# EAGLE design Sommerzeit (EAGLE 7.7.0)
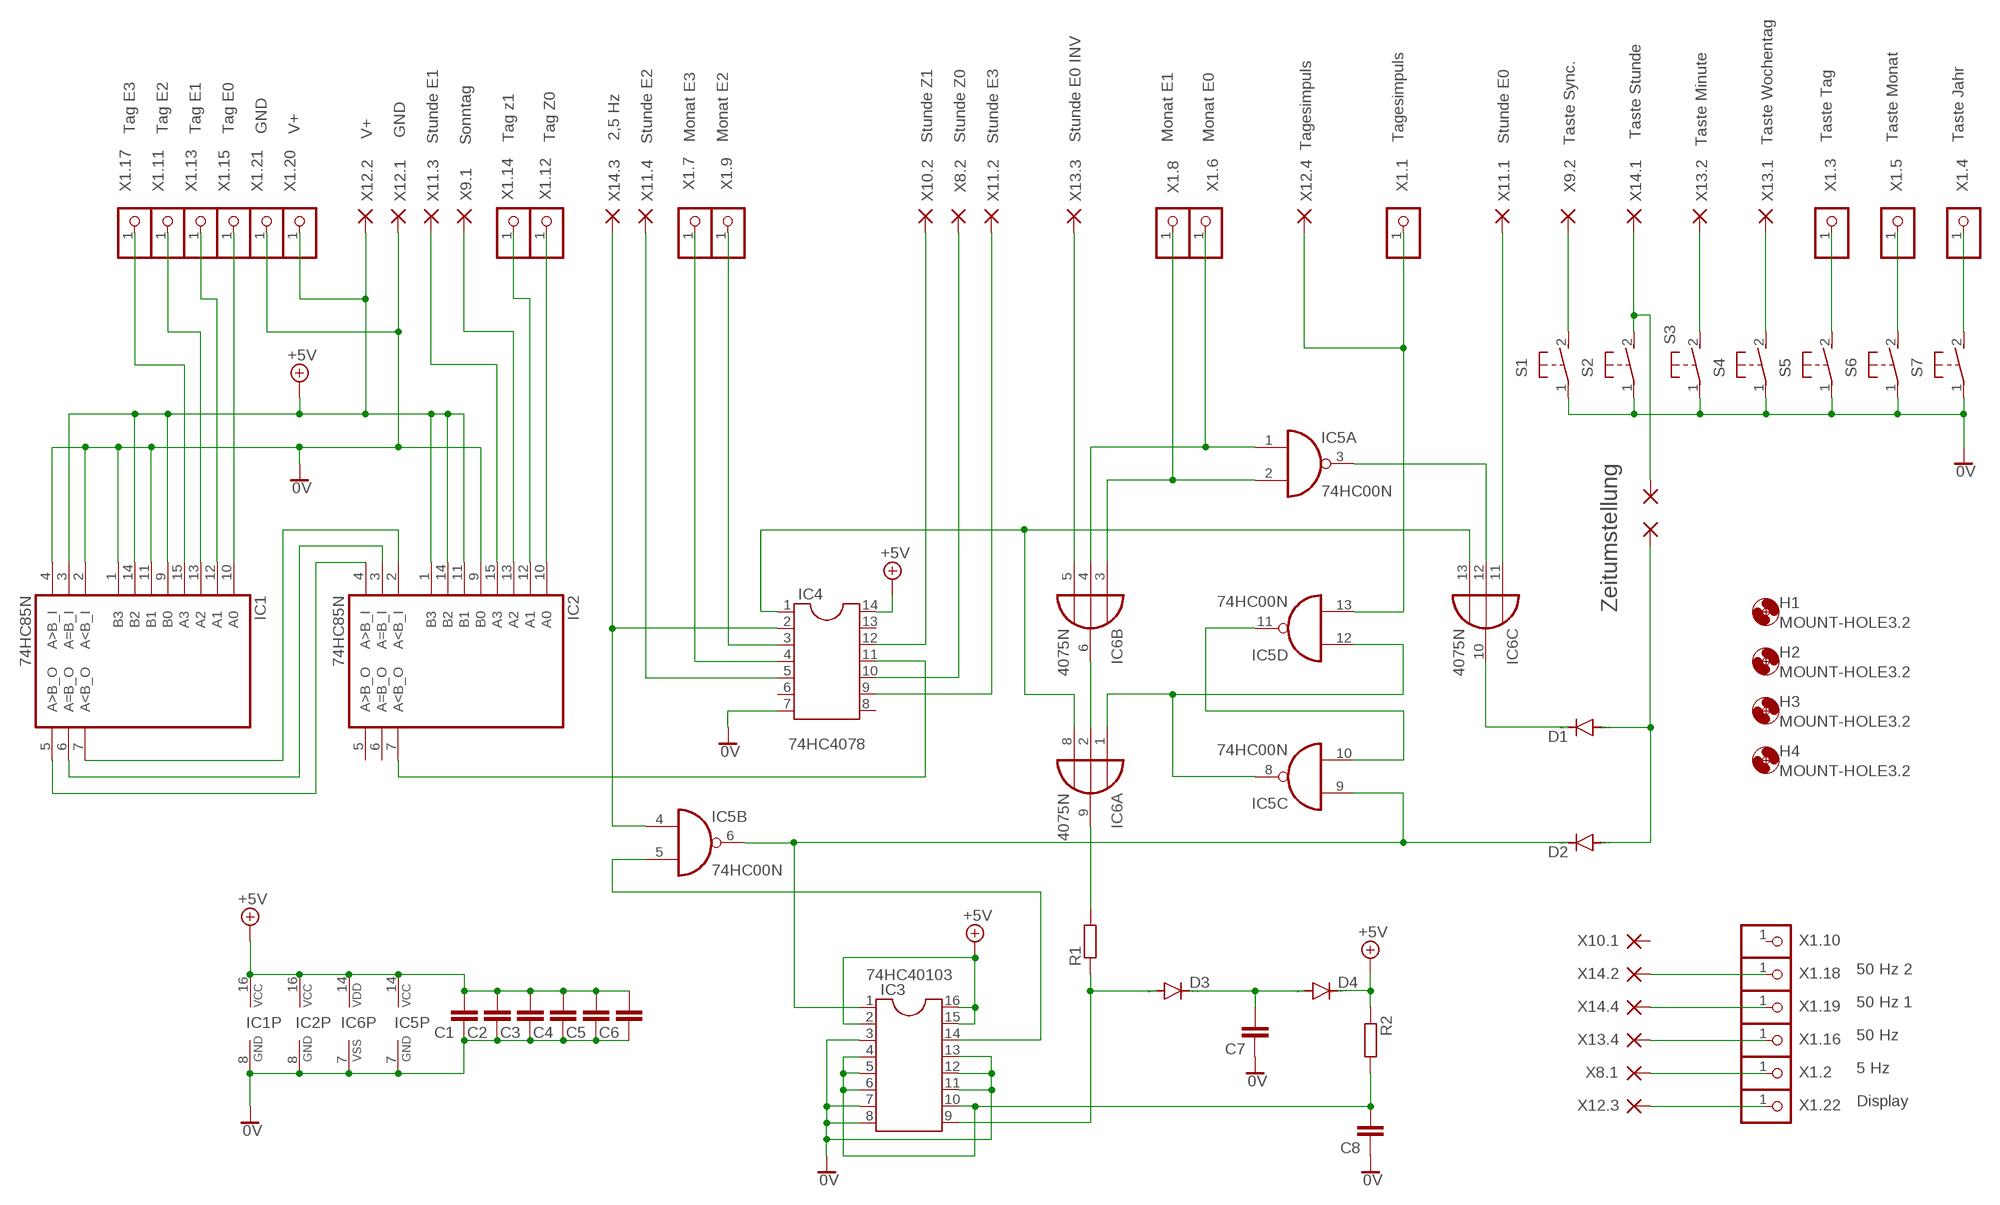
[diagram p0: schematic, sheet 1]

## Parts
C1  C-EU050-024X044  [C050-024X044]
C2  C-EU050-024X044  [C050-024X044]
C3  C-EU050-024X044  [C050-024X044]
C4  C-EU050-024X044  [C050-024X044]
C5  C-EU050-024X044  [C050-024X044]
C6  C-EU050-024X044  [C050-024X044]
C7  C-EU050-024X044  [C050-024X044]
C8  C-EU050-024X044  [C050-024X044]
D1  1N4148DO35-10  [DO35-10]
D2  1N4148DO35-10  [DO35-10]
D3  1N4148DO35-10  [DO35-10]
D4  1N4148DO35-10  [DO35-10]
H1  MOUNT-HOLE3.2  [3,2]
H2  MOUNT-HOLE3.2  [3,2]
H3  MOUNT-HOLE3.2  [3,2]
H4  MOUNT-HOLE3.2  [3,2]
IC1  74HC85N  [DIL16]
IC2  74HC85N  [DIL16]
IC3  DIL16  [DIL16]
IC4  DIL14  [DIL14]
IC5  74HC00N  [DIL14]
IC6  4075N  [DIL14]
PAD1  WIREPAD1,6/0,8  [1,6/0,8]
PAD2  WIREPAD1,6/0,8  [1,6/0,8]
R1  R-EU_0207/10  [0207/10]
R2  R-EU_0207/10  [0207/10]
S1  31-XX  [B3F-31XX]
S2  31-XX  [B3F-31XX]
S3  31-XX  [B3F-31XX]
S4  31-XX  [B3F-31XX]
S5  31-XX  [B3F-31XX]
S6  31-XX  [B3F-31XX]
S7  31-XX  [B3F-31XX]
X1.1  Tagesimpuls  PINHD-1X1  [1X01]
X1.2  5 Hz  PINHD-1X1  [1X01]
X1.3  Taste Tag  PINHD-1X1  [1X01]
X1.4  Taste Jahr  PINHD-1X1  [1X01]
X1.5  Taste Monat  PINHD-1X1  [1X01]
X1.6  Monat E0  PINHD-1X1  [1X01]
X1.7  Monat E3  PINHD-1X1  [1X01]
X1.8  Monat E1  PINHD-1X1  [1X01]
X1.9  Monat E2  PINHD-1X1  [1X01]
X1.10  PINHD-1X1  [1X01]
X1.11  Tag E2  PINHD-1X1  [1X01]
X1.12  Tag Z0  PINHD-1X1  [1X01]
X1.13  Tag E1  PINHD-1X1  [1X01]
X1.14  Tag z1  PINHD-1X1  [1X01]
X1.15  Tag E0  PINHD-1X1  [1X01]
X1.16  50 Hz  PINHD-1X1  [1X01]
X1.17  Tag E3  PINHD-1X1  [1X01]
X1.18  50 Hz 2  PINHD-1X1  [1X01]
X1.19  50 Hz 1  PINHD-1X1  [1X01]
X1.20  V+  PINHD-1X1  [1X01]
X1.21  GND  PINHD-1X1  [1X01]
X1.22  Display  PINHD-1X1  [1X01]
X8.1  WIREPAD1,6/0,8  [1,6/0,8]
X8.2  Stunde Z0  WIREPAD1,6/0,8  [1,6/0,8]
X9.1  Sonntag  WIREPAD1,6/0,8  [1,6/0,8]
X9.2  Taste Sync.  WIREPAD1,6/0,8  [1,6/0,8]
X10.1  WIREPAD1,6/0,8  [1,6/0,8]
X10.2  Stunde Z1  WIREPAD1,6/0,8  [1,6/0,8]
X11.1  Stunde E0  WIREPAD1,6/0,8  [1,6/0,8]
X11.2  Stunde E3  WIREPAD1,6/0,8  [1,6/0,8]
X11.3  Stunde E1  WIREPAD1,6/0,8  [1,6/0,8]
X11.4  Stunde E2  WIREPAD1,6/0,8  [1,6/0,8]
X12.1  GND  WIREPAD1,6/0,8  [1,6/0,8]
X12.2  V+  WIREPAD1,6/0,8  [1,6/0,8]
X12.3  WIREPAD1,6/0,8  [1,6/0,8]
X12.4  Tagesimpuls  WIREPAD1,6/0,8  [1,6/0,8]
X13.1  Taste Wochentag  WIREPAD1,6/0,8  [1,6/0,8]
X13.2  Taste Minute  WIREPAD1,6/0,8  [1,6/0,8]
X13.3  Stunde E0 INV  WIREPAD1,6/0,8  [1,6/0,8]
X13.4  WIREPAD1,6/0,8  [1,6/0,8]
X14.1  Taste Stunde  WIREPAD1,6/0,8  [1,6/0,8]
X14.2  WIREPAD1,6/0,8  [1,6/0,8]
X14.3  2,5 Hz  WIREPAD1,6/0,8  [1,6/0,8]
X14.4  WIREPAD1,6/0,8  [1,6/0,8]

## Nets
0V: C1.1 C2.1 C3.1 C4.1 C5.1 C6.1 C7.1 C8.1 IC1.1(B3) IC1.2(A<B_I) IC1.4(A>B_I) IC1.8(GND) IC1.11(B1) IC2.8(GND) IC2.9(B0) IC3.3 IC3.7 IC3.8 IC3.11 IC3.12 IC3.13 IC4.7 IC5.7(P:GND) IC6.7(P:VSS) S1.1(P) S2.1(P) S3.1(P) S4.1(P) S5.1(P) S6.1(P) S7.1(P) X1.21.1 X12.1.1(P)
+5V: C1.2 C2.2 C3.2 C4.2 C5.2 C6.2 D4.C IC1.3(A=B_I) IC1.9(B0) IC1.14(B2) IC1.16(VCC) IC2.1(B3) IC2.11(B1) IC2.14(B2) IC2.16(VCC) IC3.2 IC3.15 IC3.16 IC4.14 IC5.14(P:VCC) IC6.14(P:VDD) R2.1 X1.20.1 X12.2.1(P)
N$1: IC1.7(A<B_O) IC2.2(A<B_I)
N$2: IC1.6(A=B_O) IC2.3(A=B_I)
N$3: IC1.5(A>B_O) IC2.4(A>B_I)
N$4: IC2.7(A<B_O) IC4.11
N$5: IC4.1 IC6.8(A:I2) IC6.13(C:I2)
N$6: IC6.2(A:I1) IC6.6(B:O)
N$7: IC5.8(C:O) IC5.12(D:I0) IC6.1(A:I0)
N$8: IC5.10(C:I1) IC5.11(D:O)
N$9: IC5.13(D:I1) X1.1.1 X12.4.1(P)
N$10: IC2.10(A0) X1.12.1
N$11: IC2.12(A1) X1.14.1
N$12: IC1.10(A0) X1.15.1
N$13: IC4.12 X10.2.1(P)
N$14: IC1.12(A1) X1.13.1
N$15: IC1.13(A2) X1.11.1
N$16: IC1.15(A3) X1.17.1
N$17: IC2.15(A3) X11.3.1(P)
N$18: IC2.13(A2) X9.1.1(P)
N$19: IC4.10 X8.2.1(P)
N$20: IC4.9 X11.2.1(P)
N$21: IC4.4 X1.7.1
N$22: IC4.3 X1.9.1
N$23: IC4.5 X11.4.1(P)
N$24: IC4.2 IC5.4(B:I0) X14.3.1(P)
N$25: IC6.5(B:I2) X13.3.1(P)
N$26: IC5.1(A:I0) IC6.4(B:I1) X1.6.1
N$27: IC5.3(A:O) IC6.12(C:I1)
N$28: IC6.11(C:I0) X11.1.1(P)
N$29: IC5.2(A:I1) IC6.3(B:I0) X1.8.1
N$30: D1.C IC6.10(C:O)
N$31: PAD2.1(P) S2.2(S) X14.1.1(P)
N$32: D2.C IC3.1 IC5.6(B:O) IC5.9(C:I0)
N$34: X1.22.1 X12.3.1(P)
N$35: IC6.9(A:O) R1.2
N$36: C7.2 D3.C D4.A
N$37: X1.18.1 X14.2.1(P)
N$38: D1.A D2.A PAD1.1(P)
N$40: C8.2 IC3.4 IC3.5 IC3.6 IC3.10 R2.2
N$43: S1.2(S) X9.2.1(P)
N$44: IC3.14 IC5.5(B:I1)
N$45: S3.2(S) X13.2.1(P)
N$46: S4.2(S) X13.1.1(P)
N$47: S5.2(S) X1.3.1
N$48: S6.2(S) X1.5.1
N$49: S7.2(S) X1.4.1
N$50: D3.A IC3.9 R1.1
N$51: X1.19.1 X14.4.1(P)
N$52: X1.16.1 X13.4.1(P)
N$53: X1.2.1 X8.1.1(P)
Unconnected: IC2.5(A>B_O) IC2.6(A=B_O) IC4.6 IC4.8 IC4.13 X1.10.1 X10.1.1(P)

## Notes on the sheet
- Zeitumstellung
- 74HC4078
- 74HC40103

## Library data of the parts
C1-C8 = rclxrund:C-EU: CAPACITOR, European symbol; SPICEPREFIX: C
D1-D4 = diodexrund:1N4148: DIODE
H1-H4 = holes:MOUNT-HOLE: MOUNTING HOLE with drill center marker
IC1 IC2 = 74xx-eu:74*85: 4-bit magnitude COMPARATOR
IC3 = ic-packagexrund:DIL16: Dual In Line / Socket
IC4 = ic-packagexrund:DIL14: Dual In Line / Socket
IC5 = 74xx-eu:74*00: Quad 2-input NAND gate
IC6 = 40xxrund:4075: Triple 3-input OR
PAD1 PAD2 X8.1 X8.2 X9.1 X9.2 X10.1 X10.2 X11.1-X11.4 X12.1-X12.4 X13.1-X13.4 X14.1-X14.4 = wirepad:WIREPAD: Wire PAD connect wire on PCB
R1 R2 = rclxrund:R-EU_: RESISTOR, European symbol; SPICEPREFIX: R
S1-S7 = switch-omronxrund:31-XX: OMRON SWITCH; MPN: B3F-3100; OC_FARNELL: 959704; OC_NEWARK: 36M3582
X1.1-X1.22 = pinheadxrund:PINHD-1X1: PIN HEADER

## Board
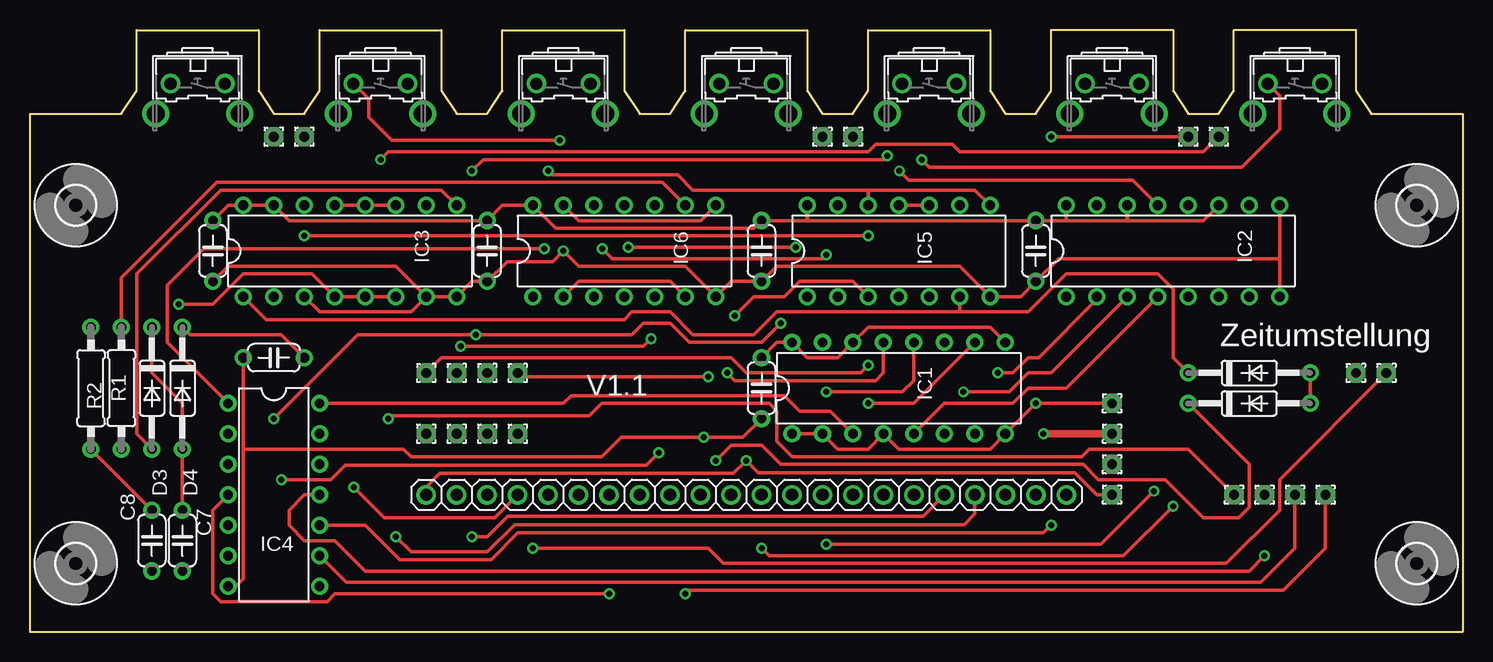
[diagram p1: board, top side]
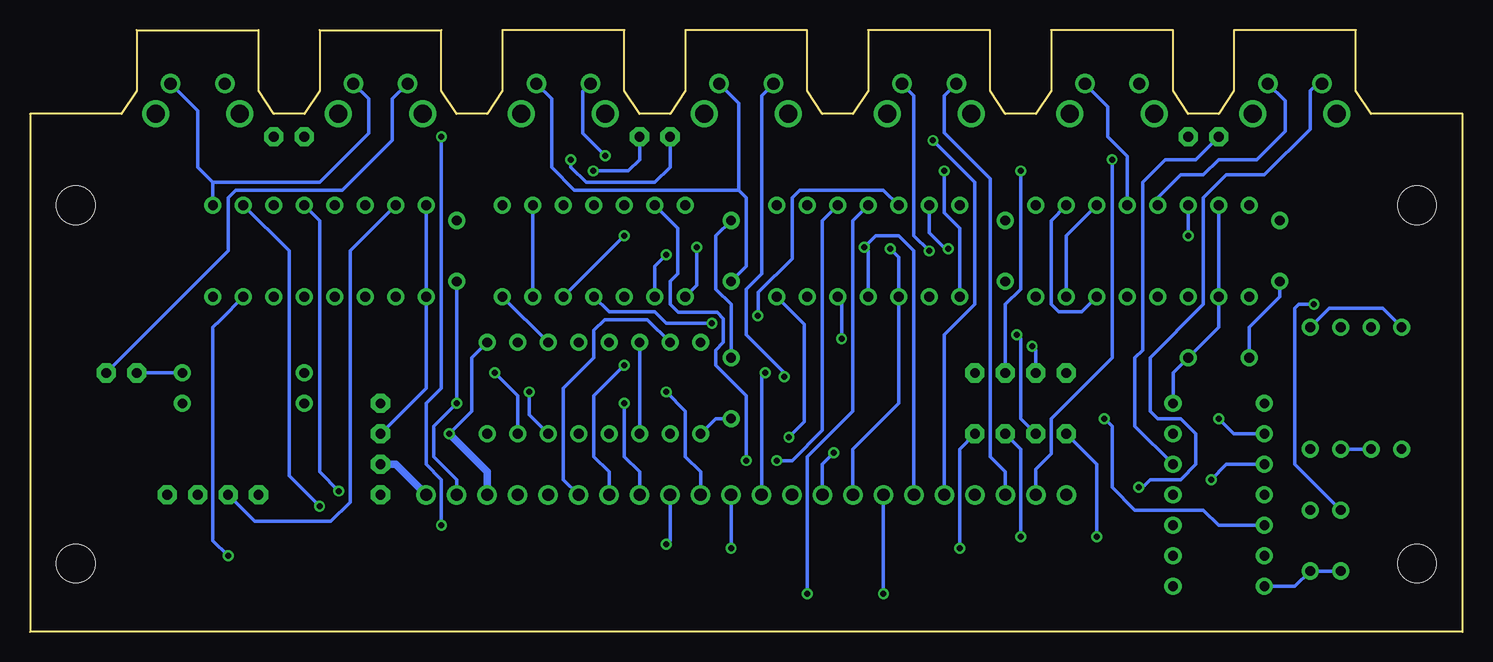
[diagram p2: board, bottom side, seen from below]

Size 119.38 x 50.16 mm. Coordinates in mm from the lower left corner, seen from the top.
Outline: 0,43.18 7.62,43.18 8.89,45.09 8.89,50.16 19.05,50.16 19.05,45.09 20.32,43.18 22.86,43.18 24.13,45.09 24.13,50.16 34.29,50.16 34.29,45.09 35.56,43.18 38.1,43.18 39.37,45.09 39.37,50.16 49.53,50.16 49.53,45.09 50.8,43.18 53.34,43.18 54.61,45.09 54.61,50.16 64.77,50.16 64.77,45.09 66.04,43.18 68.58,43.18 69.85,45.09 69.85,50.16 80.01,50.16 80.01,45.09 81.28,43.18 83.82,43.18 85.09,45.09 85.09,50.16 95.25,50.16 95.25,45.09 96.52,43.18 99.06,43.18 100.33,45.09 100.33,50.16 110.49,50.16 110.49,45.09 111.76,43.18 119.38,43.18 119.38,0 0,0 0,43.18
Copper layers (1*16): Top 0.035mm / dielectric 1.5mm / Bottom 0.035mm
Design rules "12mil *": minimum track width 12mil, minimum drill 0.5mm, track to track 12mil, track to pad 12mil, pad to pad 12mil, via to via 24mil, smd to smd 6mil, copper to edge 40mil, drill to drill 12mil, minimum pad ring 12mil, minimum via ring 8mil, stop-mask expansion 4mil, vias tented up to drill 0mil, thermal gap 10mil

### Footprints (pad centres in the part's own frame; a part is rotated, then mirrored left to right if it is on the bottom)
C050-024X044 = drill 0.813: 1 -2.54,0; 2 2.54,0
DO35-10 = drill 0.813: A 5.08,0; C -5.08,0
3,2 = hole 3.2: 0,0
DIL16 = drill 0.813: 1 -8.89,-3.81; 2 -6.35,-3.81; 3 -3.81,-3.81; 4 -1.27,-3.81; 5 1.27,-3.81; 6 3.81,-3.81; 7 6.35,-3.81; 8 8.89,-3.81; 9 8.89,3.81; 10 6.35,3.81; 11 3.81,3.81; 12 1.27,3.81; 13 -1.27,3.81; 14 -3.81,3.81; 15 -6.35,3.81; 16 -8.89,3.81
DIL14 = drill 0.813: 1 -7.62,-3.81; 2 -5.08,-3.81; 3 -2.54,-3.81; 4 0,-3.81; 5 2.54,-3.81; 6 5.08,-3.81; 7 7.62,-3.81; 8 7.62,3.81; 9 5.08,3.81; 10 2.54,3.81; 11 0,3.81; 12 -2.54,3.81; 13 -5.08,3.81; 14 -7.62,3.81
1,6/0,8 = drill 0.813 pad 1.6 octagon: 1 0,0
0207/10 = drill 0.813: 1 -5.08,0; 2 5.08,0
B3F-31XX = drill 1.016: 1 -2.261,-1.245; 2 2.261,-1.245 | drill 1.499 pad 2.159: 3 -3.505,1.245; 4 3.505,1.245
1X01 = drill 1.016: 1 0,0

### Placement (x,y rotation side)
C1  15.24,31.75 90 top
C2  38.1,31.75 90 top
C3  60.96,31.75 90 top
C4  83.82,31.75 90 top
C5  60.96,20.32 90 top
C6  20.32,22.86 0 top
C7  12.7,7.62 90 top
C8  10.16,7.62 90 top
D1  101.6,19.05 0 top
D2  101.6,21.59 0 top
D3  10.16,20.32 270 top
D4  12.7,20.32 270 top
H1  3.81,5.71 0 top
H2  3.81,35.56 0 top
H3  115.57,35.56 0 top
H4  115.57,5.71 0 top
IC1  72.39,20.32 0 top
IC2  95.25,31.75 0 top
IC3  26.67,31.75 0 top
IC4  20.32,11.43 270 top
IC5  72.39,31.75 0 top
IC6  49.53,31.75 0 top
PAD1  110.49,21.59 0 top
PAD2  113.03,21.59 0 top
R1  7.62,20.32 90 top
R2  5.08,20.32 270 top
S1  105.41,44.45 180 top
S2  90.17,44.45 180 top
S3  74.93,44.45 180 top
S4  59.69,44.45 180 top
S5  44.45,44.45 180 top
S6  29.21,44.45 180 top
S7  13.97,44.45 180 top
X1.1  33.02,11.43 0 top
X1.2  35.56,11.43 0 top
X1.3  38.1,11.43 0 top
X1.4  40.64,11.43 0 top
X1.5  43.18,11.43 0 top
X1.6  45.72,11.43 0 top
X1.7  48.26,11.43 0 top
X1.8  50.8,11.43 0 top
X1.9  53.34,11.43 0 top
X1.10  55.88,11.43 0 top
X1.11  58.42,11.43 0 top
X1.12  60.96,11.43 0 top
X1.13  63.5,11.43 0 top
X1.14  66.04,11.43 0 top
X1.15  68.58,11.43 0 top
X1.16  71.12,11.43 0 top
X1.17  73.66,11.43 0 top
X1.18  76.2,11.43 0 top
X1.19  78.74,11.43 0 top
X1.20  81.28,11.43 0 top
X1.21  83.82,11.43 0 top
X1.22  86.36,11.43 0 top
X8.1  99.06,41.27 0 top
X8.2  96.52,41.27 0 top
X9.1  68.58,41.27 0 top
X9.2  66.04,41.27 0 top
X10.1  22.86,41.27 0 top
X10.2  20.32,41.27 0 top
X11.1  107.95,11.43 0 top
X11.2  105.41,11.43 0 top
X11.3  102.87,11.43 0 top
X11.4  100.33,11.43 0 top
X12.1  90.17,19.05 0 top
X12.2  90.17,16.51 0 top
X12.3  90.17,13.97 0 top
X12.4  90.17,11.43 0 top
X13.1  40.64,21.59 0 top
X13.2  38.1,21.59 0 top
X13.3  35.56,21.59 0 top
X13.4  33.02,21.59 0 top
X14.1  40.64,16.51 0 top
X14.2  38.1,16.51 0 top
X14.3  35.56,16.51 0 top
X14.4  33.02,16.51 0 top

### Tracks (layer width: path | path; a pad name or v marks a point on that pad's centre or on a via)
0V  (via drill 0.5)
  Top 0.305: C1.1 16.51,30.48 30.48,30.48 IC3.7 | 104.14,31.11 85.72,31.11 C4.1 82.55,27.94 IC5.7 77.47,30.48 62.23,30.48 C3.1 58.42,29.21 IC6.7 54.61,30.48 45.72,30.48 v44.45,31.75 43.56,30.86 39.75,30.86 C2.1 36.83,29.21 IC3.8 IC3.7 | 104.14,31.11 IC2.8 | C6.1 17.78,15.24 | 17.78,15.24 17.78,4.45 17.14,3.81 IC4.7 | 104.14,31.11 IC2.9 | IC3.13 IC3.12 IC3.11 | IC1.1 IC1.2 67.31,15.24 69.85,15.24 IC1.4 72.39,15.24 80.01,15.24 IC1.8 v83.82,19.05 X12.1.1 | 17.78,15.24 31.11,15.24 31.75,14.61 47.62,14.61 49.26,16.23 v56.13,16.23 59.41,16.23 C5.1 | IC3.7 31.75,26.67 24.13,26.67 IC3.3
  Bottom 0.305: C4.1 v83.82,19.05 85.72,17.14 85.72,14.61 83.82,12.7 X1.21.1 | IC5.7 IC1.11 | C3.1 59.69,30.48 59.69,36.2 60.33,36.83 | C6.1 17.78,25.4 15.24,27.94 C1.1 | C8.1 C7.1 13.97,3.81 IC4.7 | v44.45,31.75 45.72,33.02 45.72,44.7 S5.1 | S4.1 60.33,44.07 60.33,36.83 | S3.1 75.92,44.42 75.92,38.71 74.04,36.83 60.33,36.83 | 104.14,37.47 95.25,37.47 91.16,41.55 91.16,44.42 S2.1 | IC2.9 104.14,37.47 | C5.1 62.23,17.78 IC1.1 | IC6.7 54.86,25.65 54.86,17.5 v56.13,16.23 | IC3.11 33.02,33.02 IC3.7 | S7.1 14.8,44.26 14.8,41.72 17.14,39.37 20.32,39.37 21.59,38.1 23.5,38.1 25.4,36.2 IC3.13 | S6.1 29.57,43.79 29.57,41.25 27.94,39.62 IC3.12 | 104.14,37.47 105.41,38.73 105.41,43.43 S1.1
+5V  (via drill 0.5)
  Top 0.305: D4.C 13.34,24.77 20.95,24.77 C6.2 | C1.2 16.51,35.56 IC3.16 IC3.15 21.59,34.29 C2.2 39.37,35.56 IC6.14 43.81,33.66 60.33,33.66 C3.2 64.77,34.29 | C4.2 86.36,34.29 IC2.16 | 91.44,34.29 IC2.14 | C4.2 91.44,34.29 | IC2.11 97.79,34.29 91.44,34.29 | C5.2 62.23,24.13 IC1.16 64.77,22.86 67.31,22.86 IC1.14 69.85,25.4 80.01,25.4 IC1.9 | 64.77,34.29 C4.2 | IC5.14 64.77,34.29 | IC1.3 66.67,18.41 64.14,18.41 62.87,19.68 45.09,19.68 44.45,19.05 IC4.14
  Top 0.61: v84.45,16.51 X12.2.1
  Bottom 0.305: IC4.14 24.13,21.59 C6.2 20.32,25.4 IC3.2 IC3.15 | IC2.16 IC2.1 86.36,20.32 X12.2.1 | IC1.14 IC1.3 | v84.45,16.51 82.55,18.41 82.55,22.86 IC1.9 | C3.2 62.23,33.02 62.23,28.57 60.96,27.3 C5.2 | R2.1 6.67,26.99 11.11,26.99 D4.C
  Bottom 0.61: v84.45,16.51 81.28,13.34 X1.20.1
N$1  (via drill 0.5)
  Top 0.305: v80.64,21.59 81.92,21.59 83.19,22.86 84.05,22.86 88.9,27.71 IC2.2
  Bottom 0.305: IC1.7 78.74,19.68 v80.64,21.59
N$2  (via drill 0.5)
  Top 0.305: v77.79,20 81.6,20 83.19,21.59 85.09,21.59 IC2.3
  Bottom 0.305: IC1.6 77.79,18.1 v77.79,20
N$3
  Top 0.305: IC1.5 76.2,19.05 81.92,19.05 83.19,20.32 86.36,20.32 IC2.4
N$4  (via drill 0.5)
  Top 0.305: v102.87,6.35 101.6,5.08 27.94,5.08 25.4,7.62 22.86,7.62 21.59,8.89 21.59,10.16 22.86,11.43 IC4.11
  Bottom 0.305: v102.87,6.35 104.14,7.62 104.14,25.4 103.5,26.04 IC2.7
N$5  (via drill 0.5)
  Top 0.305: IC4.1 11.43,24.13 11.43,28.89 14.48,31.94 v42.86,31.94 | IC6.8 55.88,34.29 45.72,34.29 IC6.13
  Bottom 0.305: v42.86,31.94 43.12,31.94 44.45,33.27 IC6.13
N$6
  Top 0.305: IC6.2 45.72,29.21 53.34,29.21 IC6.6
N$7  (via drill 0.5)
  Top 0.305: v43.18,38.42 43.5,38.1 53.98,38.1 55.24,36.83 69.85,36.83 | IC5.12 69.85,36.83 | IC5.8 78.74,36.83 69.85,36.83
  Bottom 0.305: IC6.1 41.91,33.66 43.18,34.92 v43.18,38.42
N$8
  Top 0.305: IC5.10 IC5.11
N$9  (via drill 0.5)
  Top 0.305: X1.1.1 33.02,12.06 34.16,13.21 58.61,13.21 v59.69,14.29 60.71,13.27 87.06,13.27 88.9,11.43 X12.4.1
  Bottom 0.305: v59.69,14.29 59.69,19.68 62.23,22.23 62.23,23.5 61.59,24.13 61.59,26.1 62.12,26.63 65.36,26.63 66.04,27.3 66.04,29.21 65.41,29.84 65.41,33.66 IC5.13
N$10  (via drill 0.5)
  Top 0.305: v95.25,10.48 91.12,6.35 61.59,6.35 v60.96,6.99
  Bottom 0.305: IC2.10 97.79,31.75 97.79,13.02 v95.25,10.48 | X1.12.1 v60.96,6.99
N$11  (via drill 0.5)
  Top 0.305: v93.66,11.75 89.22,7.3 v66.36,7.3
  Bottom 0.305: IC2.12 95.25,34.29 95.25,13.34 v93.66,11.75 | X1.14.1 66.04,7.62 v66.36,7.3
N$12  (via drill 0.5)
  Top 0.305: IC1.10 73.66,19.05 v69.85,19.05
  Bottom 0.305: X1.15.1 68.58,13.34 69.85,14.61 v69.85,19.05
N$13
  Bottom 0.305: IC4.12 27.3,17.14 27.3,22.86 26.67,23.5 26.67,37.47 24.77,39.37 22.23,39.37 X10.2.1
N$14  (via drill 0.5)
  Top 0.305: IC1.12 73.66,20.95 72.71,20 v66.36,20
  Bottom 0.305: v66.36,20 64.77,18.41 64.77,14.61 63.5,13.34 X1.13.1
N$15  (via drill 0.5)
  Top 0.305: IC1.13 71.12,21.59 70.48,20.95 58.74,20.95 v58.1,21.59
  Bottom 0.305: v58.1,21.59 58.42,21.27 X1.11.1
N$16
  Bottom 0.305: IC1.15 67.94,26.04 71.5,26.04 72.39,25.15 72.39,22.86 74.93,20.32 74.93,12.7 X1.17.1
N$17
  Bottom 0.305: IC2.15 92.71,31.75 92.71,10.79 94.3,9.21 100.65,9.21 X11.3.1
N$18  (via drill 0.5)
  Top 0.305: v72.45,38.42 73.22,37.66 91.89,37.66 IC2.13
  Bottom 0.305: X9.1.1 68.58,39.37 69.53,38.42 v72.45,38.42
N$19  (via drill 0.5)
  Top 0.305: IC4.10 27.94,8.89 30.8,6.03 38.42,6.03 40.64,8.26 84.45,8.26 v85.09,8.89 | v85.09,41.27 X8.2.1
  Bottom 0.305: v85.09,8.89 85.09,12.7 86.36,13.97 86.36,19.05 85.09,20.32 v85.09,41.27
N$20
  Top 0.305: IC4.9 26.35,4.13 102.55,4.13 105.41,6.99 X11.2.1
N$21  (via drill 0.5)
  Top 0.305: IC4.4 15.24,10.16 15.24,3.17 15.88,2.54 24.77,2.54 25.4,3.17 v48.26,3.17
  Bottom 0.305: X1.7.1 v48.26,3.17
N$22  (via drill 0.5)
  Top 0.305: v20.95,12.7 25.08,12.7 26.29,13.91 51.37,13.91 v52.39,14.92
  Bottom 0.305: v20.95,12.7 19.68,13.97 IC4.3 | X1.9.1 53.34,13.97 v52.39,14.92
N$23  (via drill 0.5)
  Top 0.305: X11.4.1 96.52,15.24 88.27,15.24 87.63,14.61 63.5,14.61 62.23,15.88 62.23,18.41 61.59,19.05 47.62,19.05 46.61,18.03 30.1,18.03 v29.84,17.78
  Bottom 0.305: v29.84,17.78 29.21,17.14 29.21,12.06 27.3,10.16 21.59,10.16 20.32,8.89 IC4.5
N$24  (via drill 0.5)
  Top 0.305: v62.55,25.72 60.96,24.13 54.93,24.13 53.34,25.72 51.12,25.72 50.16,24.77 v37.15,24.77 27.3,24.77 v20.32,17.78
  Bottom 0.305: IC5.4 71.12,26.67 67.31,26.67 66.36,25.72 v62.55,25.72 | v37.15,24.77 36.83,24.45 36.83,17.78 X14.3.1 | v20.32,17.78 19.05,16.51 IC4.2
N$25  (via drill 0.5)
  Top 0.305: v51.75,24.45 51.12,23.81 v35.88,23.81
  Bottom 0.305: IC6.5 51.75,27.62 v51.75,24.45 | v35.88,23.81 35.56,23.5 X13.3.1
N$26  (via drill 0.5)
  Top 0.305: v49.85,32.07 v63.82,32.07
  Bottom 0.305: X1.6.1 45.72,31.75 46.99,33.02 48.9,33.02 v49.85,32.07 49.53,31.75 IC6.4 | IC5.1 63.82,28.89 v63.82,32.07
N$27  (via drill 0.5)
  Top 0.305: v58.74,26.35 60.33,27.94 62.87,27.94 64.14,29.21 68.58,29.21 IC5.3
  Bottom 0.305: IC6.12 48.26,36.83 55.24,36.83 55.88,36.2 55.88,31.11 58.67,28.32 58.67,26.42 v58.74,26.35
N$28  (via drill 0.5)
  Top 0.305: v54.61,3.17 54.93,3.49 104.46,3.49 107.95,6.99 X11.1.1
  Bottom 0.305: IC6.11 50.8,34.29 50.8,18.41 54.61,14.61 v54.61,3.17
N$29  (via drill 0.5)
  Top 0.305: v66.36,31.43 66.04,31.11 48.51,31.11 v47.69,31.94
  Bottom 0.305: X1.8.1 50.8,15.24 46.99,19.05 IC6.3 46.99,31.24 v47.69,31.94 | v66.36,31.43 67.31,30.48 IC5.2
N$30  (via drill 0.5)
  Top 0.305: v57.15,14.29 58.42,15.56 60.96,15.56 62.55,13.97 87.76,13.97 89.03,12.7 94.61,12.7 97.79,9.53 100.71,9.53 101.6,10.41 101.6,13.97 D1.C
  Bottom 0.305: IC6.10 53.34,34.29 53.34,16.83 55.88,14.29 v57.15,14.29
N$31  (via drill 0.5)
  Top 0.305: v41.91,6.99 56.52,6.99 57.78,5.71 99.69,5.71 104.14,10.16 104.14,12.7 PAD2.1
  Bottom 0.305: X14.1.1 41.91,15.24 v41.91,6.99 | S2.2 89.18,44.42 89.18,41 93.34,36.83 102.23,36.83 102.87,36.2 102.87,31.75 PAD2.1
N$32
  Top 0.305: IC3.1 19.68,26.04 49.53,26.04 50.16,26.67 53.34,26.67 55.24,24.77 60.31,24.77 62.21,26.67 77.47,26.67 | IC5.6 77.47,26.67 | 77.47,26.67 83.19,26.67 86.36,29.84 93.98,29.84 95.25,28.57 95.25,22.86 D2.C
  Bottom 0.305: IC5.6 IC5.9
N$34
  Bottom 0.61: X1.22.1 88.9,13.97 X12.3.1
N$35
  Top 0.305: R1.2 7.62,29.53 15.56,37.47 52.7,37.47 IC6.9
N$36
  Top 0.305: D3.C 10.16,21.59 12.7,19.05 D4.A C7.2
N$37  (via drill 0.5)
  Top 0.305: v36.83,7.94 38.1,7.94 39.81,9.65 74.42,9.65 X1.18.1
  Bottom 0.305: X14.2.1 36.83,15.24 v36.83,7.94
N$38
  Top 0.305: D1.A D2.A
  Bottom 0.305: PAD1.1 D2.A
N$40  (via drill 0.5)
  Top 0.305: IC3.6 IC3.5 IC3.4 23.5,29.84 17.78,29.84 15.24,27.3 v12.38,27.3 | C8.2 R2.2
  Bottom 0.305: IC3.10 34.29,34.29 34.29,27.3 33.66,26.67 31.75,26.67 IC3.6 | v12.38,27.3 13.65,27.3 13.97,26.99 13.97,13.97 C8.2
N$43  (via drill 0.5)
  Top 0.305: S1.2 104.14,44.7 104.14,41.91 100.97,38.73 74.93,38.73 v74.3,39.36
  Bottom 0.305: v74.3,39.36 74.3,38.74 73.03,37.47 67.31,37.47 66.04,38.73 X9.2.1
N$44  (via drill 0.5)
  Top 0.305: v69.85,33.02 v22.86,33.02
  Bottom 0.305: v22.86,33.02 IC3.14 | IC5.5 v69.85,33.02
N$45  (via drill 0.5)
  Top 0.305: v36.83,38.42 37.78,39.37 71.12,39.37 v71.44,39.69
  Bottom 0.305: X13.2.1 38.1,27.3 36.83,28.57 v36.83,38.42 | v71.44,39.69 73.3,41.55 73.3,45.06 S3.2
N$46  (via drill 0.5)
  Top 0.305: X13.1.1 40.96,21.27 v56.52,21.27
  Bottom 0.305: S4.2 58.42,44.7 58.42,29.84 59.69,28.57 59.69,24.77 56.52,21.59 v56.52,21.27
N$47
  Bottom 0.305: X1.3.1 38.1,13.34 39.37,14.61 39.37,37.78 43.18,41.59 43.18,44.7 S5.2
N$48  (via drill 0.5)
  Top 0.305: S6.2 28.22,44.42 28.22,42.9 30.16,40.96 v44.13,40.96
  Bottom 0.305: X1.5.1 43.18,24.77 40.64,27.3 40.64,37.47 v44.13,40.96
N$49  (via drill 0.5)
  Top 0.305: X1.4.1 38.73,9.53 29.53,9.53 v26.99,12.06
  Bottom 0.305: S7.2 12.1,45.3 12.15,45.64 12.7,45.09 12.7,41.91 16.51,38.1 19.68,38.1 21.59,36.2 21.59,27.3 26.04,22.86 26.04,18.41 25.4,17.78 23.5,17.78 22.23,16.51 22.23,13.97 23.5,12.7 26.04,12.7 26.67,12.06 v26.99,12.06
N$50
  Top 0.305: IC3.9 34.29,36.83 15.88,36.83 8.89,29.84 8.89,16.51 D3.A
  Bottom 0.305: D3.A R1.1
N$51  (via drill 0.5)
  Top 0.305: v30.48,7.94 31.75,6.67 38.1,6.67 40.39,8.95 77.85,8.95 78.74,9.84 X1.19.1
  Bottom 0.305: X14.4.1 30.48,13.97 v30.48,7.94
N$52  (via drill 0.5)
  Top 0.305: X13.4.1 34.29,22.86 58.42,22.86 59.69,21.59 69.22,21.59 v69.85,22.23
  Bottom 0.305: v69.85,22.23 72.39,19.68 72.39,14.61 71.12,13.34 X1.16.1
N$53  (via drill 0.5)
  Top 0.305: v29.21,39.37 29.84,40.01 69.85,40.01 70.48,40.64 76.83,40.64 77.47,40.01 97.79,40.01 X8.1.1
  Bottom 0.305: X1.2.1 35.56,13.56 34.29,14.83 34.29,17.78 29.21,22.86 v29.21,39.37

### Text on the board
tNames: Zeitumstellung | V1.1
